FUNCTION_BLOCK random_time
VAR_INPUT
	start		:	BOOL;
	Seed		:	INT:=500;
	stop		:	BOOL;

END_VAR

VAR_OUTPUT
	invisible	:	ARRAY[1..6] OF BOOL;
	buffer		:	ARRAY[0..65535]OF TIME;
	PT			:	ARRAY[1..3] OF TIME;
	Busy: BOOL;
	Done: BOOL;
END_VAR
VAR
	DRAND1		:	DRAND;
	Num			:	LREAL;
	data		:	LREAL;
	rtirg1		:	r_TRIG;
	rtirg2		:	r_TRIG;
	counter		:	UINT;
	state		:	INT;
	i			:	INT;
END_VAR


CASE state OF
	0: 	
		Busy:=FALSE;
		done:=FALSE;
		state:=1;

	1: 
		Busy:=FALSE;
		done:=FALSE;
		Rtirg1(CLK:= start, Q=> );
		IF Rtirg1.Q THEN
			Busy:=TRUE;
			state := 2;
		END_IF

	//随机数一直生成	
	2: 
		DRAND1(Seed:= Seed, Num=>Num );    (*Seed随便填，如果一个程序中使用多个DRAND，那么每个Seed就设为不同的数，产生的随机数也会不同*)
		data:=1500*Num+1000;     (* 产生一个1000ms~2500ms之间的随机整数*)
		PT[1]:=LREAL_TO_TIME(data);
		PT[2]:=LREAL_TO_TIME(data*1.5+500);
		PT[3]:=LREAL_TO_TIME(data*2+800);
		
		rtirg2(CLK:=stop , Q=> );
		
	//停止随机数并保存
		IF rtirg2.Q THEN
			IF counter < 0 OR counter > 65535 THEN
				counter:= 0;
			END_IF	  		
			buffer[counter] := PT[1];
			counter:= counter + 1;
			
			Busy:=FALSE;
			done:=TRUE;
			state:=1;
		END_IF



END_CASE

END_FUNCTION_BLOCK
